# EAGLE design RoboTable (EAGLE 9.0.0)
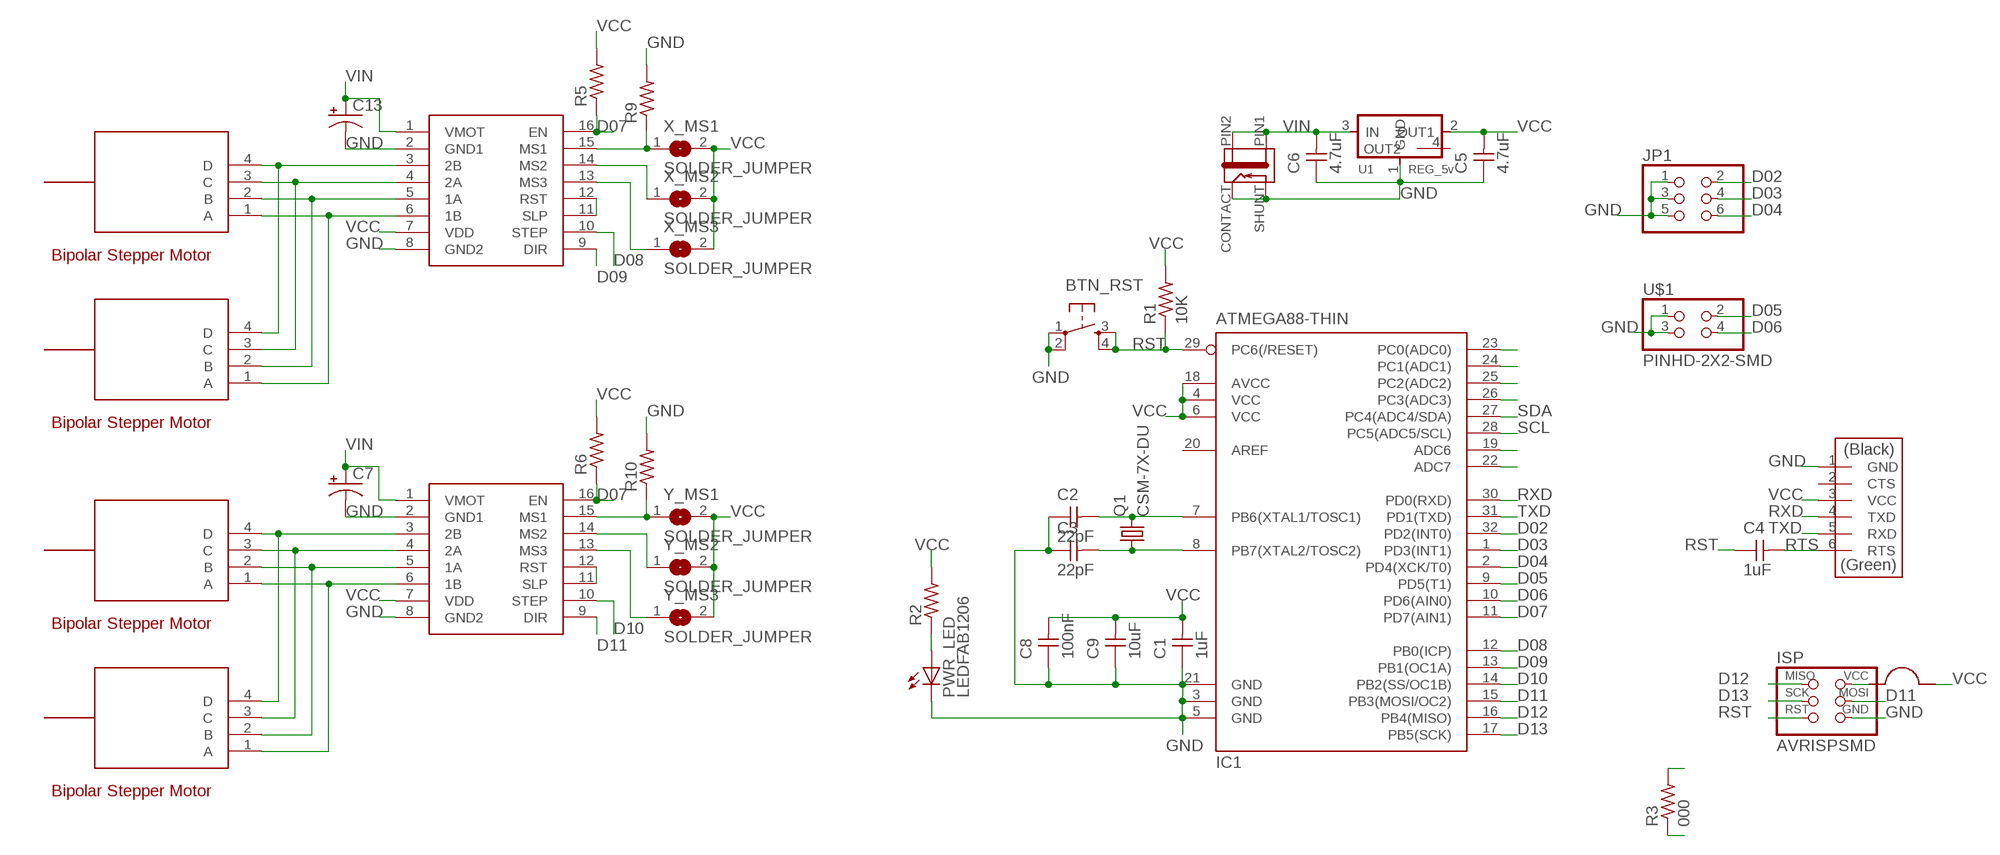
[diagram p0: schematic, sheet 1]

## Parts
BTN_RST  6MM_SWITCH  [6MM_SWITCH_2]
C1  1uF  CAP-UNPOLARIZEDFAB  [C1206FAB]
C2  22pF  CAP-UNPOLARIZEDFAB  [C1206FAB]
C3  22pF  CAP-UNPOLARIZEDFAB  [C1206FAB]
C4  1uF  CAP-UNPOLARIZEDFAB  [C1206FAB]
C5  4.7uF  CAP-UNPOLARIZEDFAB  [C1206FAB]
C6  4.7uF  CAP-UNPOLARIZEDFAB  [C1206FAB]
C7  CPOL-USC  [PANASONIC_C]
C8  100nF  CAP-UNPOLARIZEDFAB  [C1206FAB]
C9  10uF  CAP-UNPOLARIZEDFAB  [C1206FAB]
C13  CPOL-USC  [PANASONIC_C]
FTDI  FTDI-SMD-HEADER  [1X06SMD]
IC1  ATMEGA88-THIN  [TQFP32-08THIN]
ISP  AVRISPSMD  [2X03SMD]
J1  JACK-2.1MM  [PJ-002AH-SMT]
JP1  PINHD-2X3-SMD  [2X03SMD]
PWR_LED  LEDFAB1206  [LED1206FAB]
Q1  CSM-7X-DU  [CSM-7X-DU]
R1  10K  RES-US1206FAB  [R1206FAB]
R2  RES-US1206FAB  [R1206FAB]
R3  000  RES-US1206FAB  [R1206FAB]
R5  RES-US1206FAB  [R1206FAB]
R6  RES-US1206FAB  [R1206FAB]
R9  RES-US1206FAB  [R1206FAB]
R10  RES-US1206FAB  [R1206FAB]
U1  REG_5v  REGULATOR_SOT223  [SOT223]
U$1  PINHD-2X2-SMD  [2X02SMD]
U$4  JUMPER  [JUMPER]
X1_MOTOR  STEPPER_MOTORCONN_1X4  [CONN_1X4]
X2_MOTOR  STEPPER_MOTORCONN_1X4  [CONN_1X4]
X_DRIVER  POLOLUESTEPPERDRIVER  [DIL16]
X_MS1  SOLDER_JUMPER  [SJFAB]
X_MS2  SOLDER_JUMPER  [SJFAB]
X_MS3  SOLDER_JUMPER  [SJFAB]
Y1_MOTOR  STEPPER_MOTORCONN_1X4  [CONN_1X4]
Y2_MOTOR  STEPPER_MOTORCONN_1X4  [CONN_1X4]
Y_DRIVER  POLOLUESTEPPERDRIVER  [DIL16]
Y_MS1  SOLDER_JUMPER  [SJFAB]
Y_MS2  SOLDER_JUMPER  [SJFAB]
Y_MS3  SOLDER_JUMPER  [SJFAB]

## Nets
A_MS1: R9.1 X_DRIVER.15(MS1) X_MS1.1
A_MS2: X_DRIVER.14(MS2) X_MS2.1
A_MS3: X_DRIVER.13(MS3) X_MS3.1
B_MS1: R10.1 Y_DRIVER.15(MS1) Y_MS1.1
B_MS2: Y_DRIVER.14(MS2) Y_MS2.1
B_MS3: Y_DRIVER.13(MS3) Y_MS3.1
D02: IC1.32(PD2(INT0)) JP1.2
D03: IC1.1(PD3(INT1)) JP1.4
D04: IC1.2(PD4(XCK/T0)) JP1.6
D05: IC1.9(PD5(T1)) U$1.2
D06: IC1.10(PD6(AIN0)) U$1.4
D07: IC1.11(PD7(AIN1)) R5.1 R6.1 X_DRIVER.16(EN) Y_DRIVER.16(EN)
D08: IC1.12(PB0(ICP)) X_DRIVER.10(STEP)
D09: IC1.13(PB1(OC1A)) X_DRIVER.9(DIR)
D10: IC1.14(PB2(SS/OC1B)) Y_DRIVER.10(STEP)
D11: IC1.15(PB3(MOSI/OC2)) ISP.4(MOSI) Y_DRIVER.9(DIR)
D12: IC1.16(PB4(MISO)) ISP.1(MISO)
D13: IC1.17(PB5(SCK)) ISP.3(SCK)
GND: BTN_RST.1(P) BTN_RST.2(P1) C1.1 C2.1 C3.1 C5.1 C6.1 C7.- C8.1 C9.1 C13.- FTDI.1(GND) IC1.3(GND) IC1.5(GND) IC1.21(GND) ISP.6(GND) J1.CONTACT J1.SHUNT JP1.1 JP1.3 JP1.5 PWR_LED.2(C) R9.2 R10.2 U1.1(GND) U$1.1 U$1.3 X_DRIVER.2(GND1) X_DRIVER.8(GND2) Y_DRIVER.2(GND1) Y_DRIVER.8(GND2)
LED: PWR_LED.1(A) R2.1
N$1: X_DRIVER.11(SLP) X_DRIVER.12(RST)
N$2: Y_DRIVER.11(SLP) Y_DRIVER.12(RST)
N$3: IC1.23(PC0(ADC0))
N$4: IC1.24(PC1(ADC1))
N$5: IC1.25(PC2(ADC2))
N$6: IC1.26(PC3(ADC3))
N$7: IC1.19(ADC6)
N$8: IC1.22(ADC7)
RST: BTN_RST.3(S) BTN_RST.4(S1) C4.1 IC1.29(PC6(/RESET)) ISP.5(RST) R1.1 R3.1 R3.2
RTS: C4.2 FTDI.6(RTS)
RXD: FTDI.4(TXD) IC1.30(PD0(RXD))
SCL: IC1.28(PC5(ADC5/SCL))
SDA: IC1.27(PC4(ADC4/SDA))
TXD: FTDI.5(RXD) IC1.31(PD1(TXD))
VCC: C1.2 C5.2 C8.2 C9.2 FTDI.3(VCC) IC1.4(VCC) IC1.6(VCC) IC1.18(AVCC) ISP.2(VCC) R1.2 R2.2 R5.2 R6.2 U1.2(OUT1) U$4.P$1 U$4.P$2 X_DRIVER.7(VDD) X_MS1.2 X_MS2.2 X_MS3.2 Y_DRIVER.7(VDD) Y_MS1.2 Y_MS2.2 Y_MS3.2
VIN: C6.2 C7.+ C13.+ J1.PIN1 J1.PIN2 U1.3(IN) X_DRIVER.1(VMOT) Y_DRIVER.1(VMOT)
XA: X1_MOTOR.1(A) X2_MOTOR.1(A) X_DRIVER.6(1B)
XB: X1_MOTOR.2(B) X2_MOTOR.2(B) X_DRIVER.5(1A)
XC: X1_MOTOR.3(C) X2_MOTOR.3(C) X_DRIVER.4(2A)
XD: X1_MOTOR.4(D) X2_MOTOR.4(D) X_DRIVER.3(2B)
XTAL1: C2.2 IC1.7(PB6(XTAL1/TOSC1)) Q1.2
XTAL2: C3.2 IC1.8(PB7(XTAL2/TOSC2)) Q1.1
YA: Y1_MOTOR.1(A) Y2_MOTOR.1(A) Y_DRIVER.6(1B)
YB: Y1_MOTOR.2(B) Y2_MOTOR.2(B) Y_DRIVER.5(1A)
YC: Y1_MOTOR.3(C) Y2_MOTOR.3(C) Y_DRIVER.4(2A)
YD: Y1_MOTOR.4(D) Y2_MOTOR.4(D) Y_DRIVER.3(2B)
Unconnected: FTDI.2(CTS) IC1.20(AREF) U1.4(OUT2)

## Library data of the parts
BTN_RST = fab:6MM_SWITCH: OMRON SWITCH
C1-C6 C8 C9 = fab:CAP-UNPOLARIZED
C7 C13 = rcl:CPOL-US: POLARIZED CAPACITOR, American symbol; SPICEPREFIX: C
FTDI = fab:FTDI-SMD-HEADER
IC1 = fab:ATMEGA88-THIN
ISP = fab:AVRISP
J1 = fab:JACK-2.1MM: SMD DC power jack PJ-002AH-SMT As found in the fablab inventory. Made by Zaerc.
JP1 = fab:PINHD-2X3-SMD: PIN HEADER
PWR_LED = fab:LED: LED
Q1 = crystal:CSM-7X-DU: SMD CRYSTAL; OC_FARNELL: unknown; OC_NEWARK: unknown
R1-R3 R5 R6 R9 R10 = fab:RES-US: Resistor (US Symbol)
U1 = fab:REGULATOR_SOT223
U$1 = fab:PINHD-2X2-SMD
U$4 = fab:JUMPER
X1_MOTOR X2_MOTOR Y1_MOTOR Y2_MOTOR = reprap:STEPPER_MOTOR
X_DRIVER Y_DRIVER = reprap:POLOLUESTEPPERDRIVER: Pololu stepper driver based on the A4983.
X_MS1-X_MS3 Y_MS1-Y_MS3 = fab:SOLDER_JUMPER

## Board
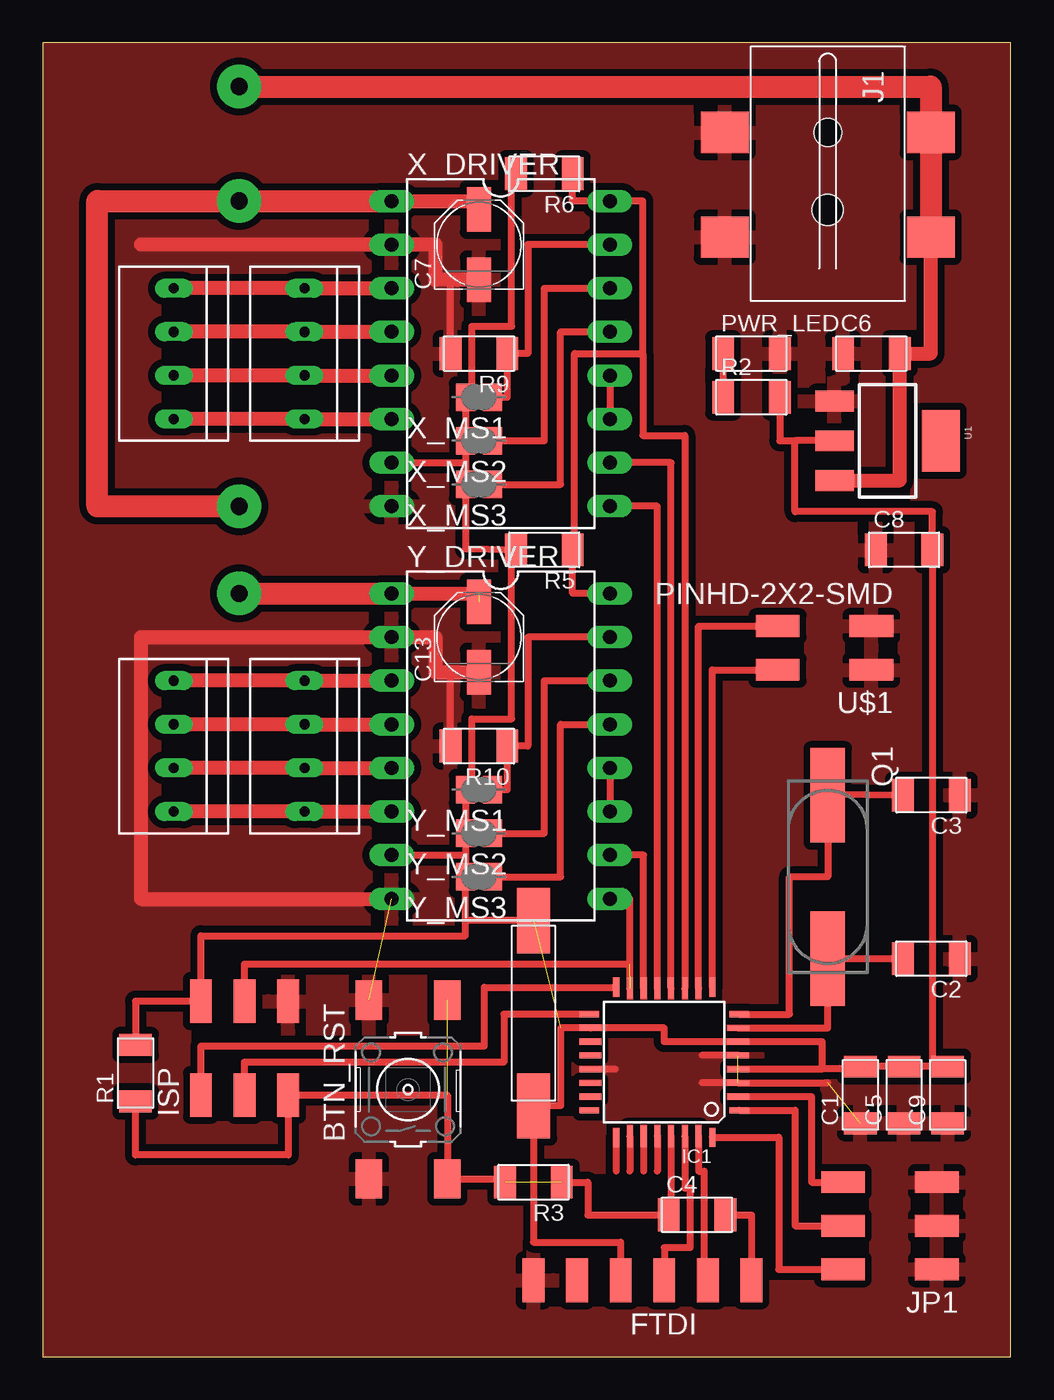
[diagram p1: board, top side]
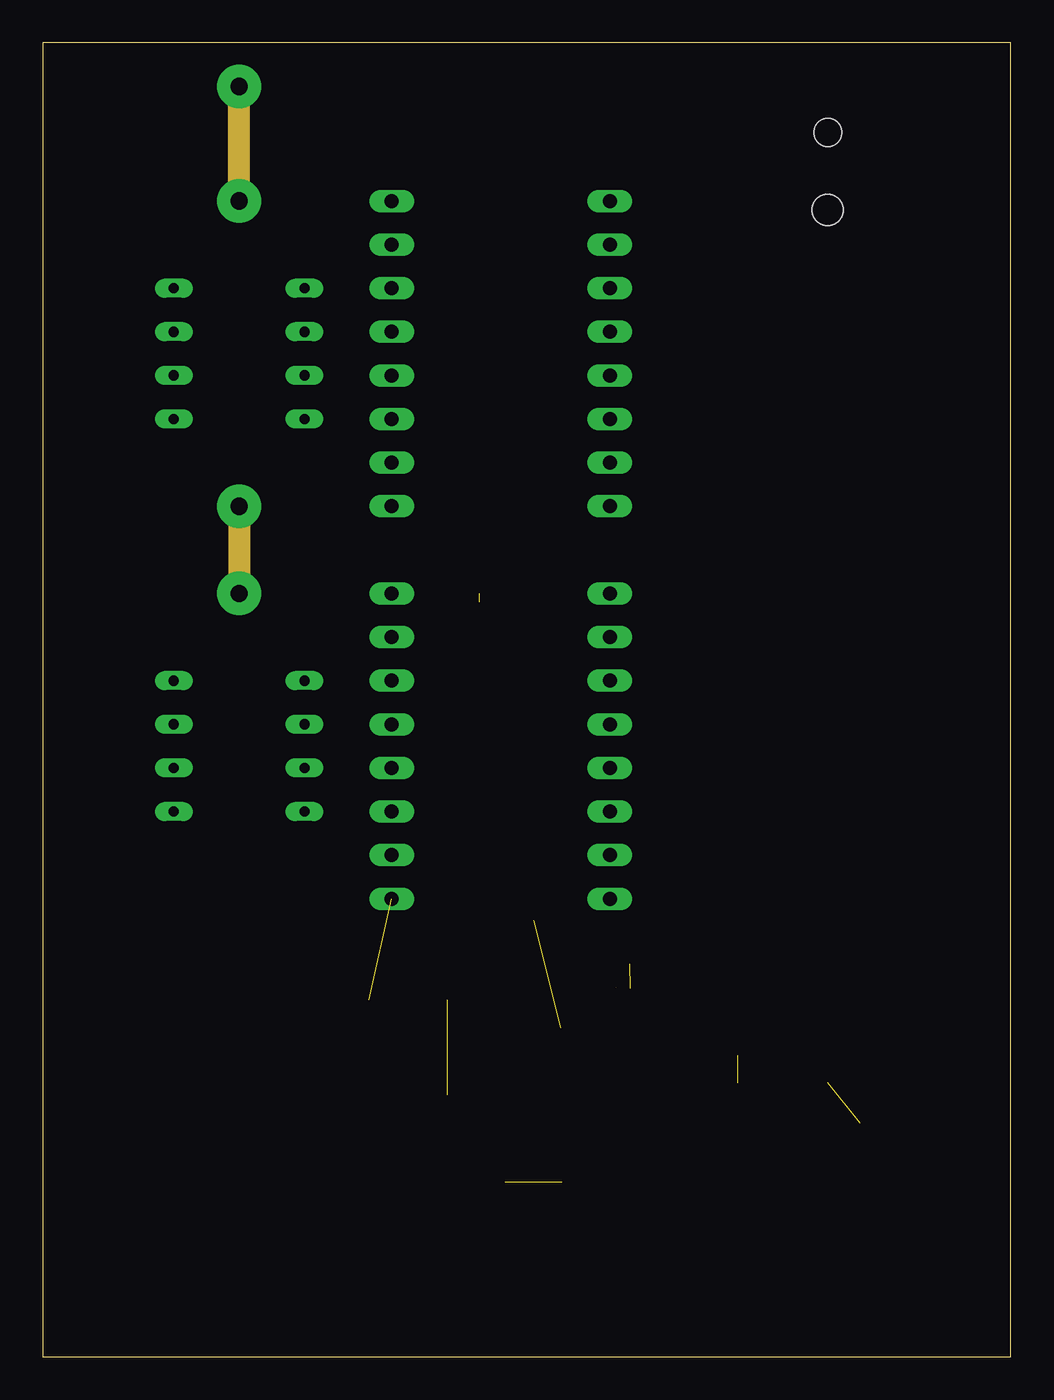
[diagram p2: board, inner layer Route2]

Size 56.39 x 76.52 mm. Coordinates in mm from the lower left corner, seen from the top.
Outline: 0,0 56.39,0 56.39,76.52 0,76.52 0,0
Copper layers (1*2): Top 0.035mm / dielectric 1.5mm / Route2 0.035mm
Design rules "default *": minimum track width 16mil, minimum drill 0.35mm, track to track 16mil, track to pad 16mil, pad to pad 16mil, via to via 16mil, smd to smd 16mil, copper to edge 1mil, drill to drill 16mil, minimum pad ring 10mil, minimum via ring 8mil, stop-mask expansion 0mil, vias tented up to drill 0mil, thermal gap 16mil

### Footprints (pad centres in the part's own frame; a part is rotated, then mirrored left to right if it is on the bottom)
6MM_SWITCH_2 = smd 2.286 x 1.524: 1 -5.207,2.286; 2 5.207,2.286; 3 -5.207,-2.286; 4 5.207,-2.286
C1206FAB = smd 1.27 x 1.905: 1 -1.651,0; 2 1.651,0
PANASONIC_C = smd 2.6 x 1.4: + 2.05,0; - -2.05,0
1X06SMD = smd 2.54 x 1.27: 1 0,6.35; 2 0,3.81; 3 0,1.27; 4 0,-1.27; 5 0,-3.81; 6 0,-6.35
TQFP32-08THIN = smd 1.118 x 0.356: 1 -4.369,2.8; 8 -4.369,-2.8; 17 4.369,-2.8; 24 4.369,2.8 | smd 1.27 x 0.356: 2 -4.293,2; 3 -4.293,1.2; 4 -4.293,0.4; 5 -4.293,-0.4; 6 -4.293,-1.2; 7 -4.293,-2; 18 4.293,-2; 19 4.293,-1.2; 20 4.293,-0.4; 21 4.293,0.4; 22 4.293,1.2; 23 4.293,2 | smd 0.356 x 1.118: 9 -2.8,-4.369; 16 2.8,-4.369; 25 2.8,4.369; 32 -2.8,4.369 | smd 0.356 x 1.27: 10 -2,-4.293; 14 1.2,-4.293; 15 2,-4.293; 26 2,4.293; 27 1.2,4.293; 31 -2,4.293 | smd 0.35 x 1.27: 11 -1.2,-4.293; 12 -0.4,-4.293; 13 0.4,-4.293; 28 0.4,4.293; 29 -0.4,4.293; 30 -1.2,4.293
2X03SMD = smd 2.54 x 1.27: 1 -2.54,2.54; 2 2.92,2.54; 3 -2.54,0; 4 2.92,0; 5 -2.54,-2.54; 6 2.92,-2.54
PJ-002AH-SMT = smd 2.4 x 2.8: CONTACT -2.4,-6; PIN1 3.7,6; PIN2 -2.4,6; SHUNT 3.7,-6 | hole 1.6: -2.4,0 | hole 1.8: 2.1,0
LED1206FAB = smd 1.27 x 1.905: 1 -1.651,0; 2 1.651,0
CSM-7X-DU = smd 5.5 x 2: 1 -4.75,0; 2 4.75,0
R1206FAB = smd 1.27 x 1.905: 1 -1.651,0; 2 1.651,0
SOT223 = smd 1.219 x 2.235: 1 -2.311,-3.099; 2 0,-3.099; 3 2.311,-3.099 | smd 3.6 x 2.2: 4 0,3.099
2X02SMD = smd 2.54 x 1.27: 1 -2.54,1.27; 2 2.92,1.27; 3 -2.54,-1.27; 4 2.92,-1.27
JUMPER = smd 3.81 x 1.93: P$1 -5.397,0; P$2 5.397,0
CONN_1X4 = drill 0.6 long: 1 -3.81,0; 2 -1.27,0; 3 1.27,0; 4 3.81,0
DIL16 = drill 0.813 long: 1 -6.35,15.24; 2 -6.35,12.7; 3 -6.35,10.16; 4 -6.35,7.62; 5 -6.35,5.08; 6 -6.35,2.54; 7 -6.35,0; 8 -6.35,-2.54; 9 6.35,-2.54; 10 6.35,0; 11 6.35,2.54; 12 6.35,5.08; 13 6.35,7.62; 14 6.35,10.16; 15 6.35,12.7; 16 6.35,15.24
SJFAB = smd 1.118 x 1.6: 1 -0.787,0; 2 0.787,0

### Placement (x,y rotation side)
BTN_RST  21.27,15.56 90 top
C1  47.62,15.24 90 top
C2  51.75,23.18 180 top
C3  51.75,32.7 180 top
C4  38.1,8.26 0 top
C5  50.16,15.24 90 top
C6  48.26,58.42 0 top
C7  25.4,64.77 90 top
C8  50.16,46.99 0 top
C9  52.7,15.24 90 top
C13  25.4,41.91 90 top
FTDI  34.92,4.45 90 top
IC1  36.2,17.14 180 top
ISP  11.75,17.78 90 top
J1  45.72,68.9 270 top
JP1  49.53,7.62 180 top
PWR_LED  41.27,58.42 0 top
Q1  45.72,27.94 270 top
R1  5.4,16.51 90 top
R2  41.27,55.88 0 top
R3  28.57,10.16 180 top
R5  29.21,46.99 180 top
R6  29.21,68.9 180 top
R9  25.4,58.42 180 top
R10  25.4,35.56 180 top
U1  49.21,53.34 270 top
U$1  45.72,41.27 180 top
U$4  28.57,20 90 top
X1_MOTOR  15.24,58.42 90 top
X2_MOTOR  7.62,58.42 90 top
X_DRIVER  26.67,52.07 0 top
X_MS1  25.4,55.88 180 top
X_MS2  25.4,53.34 180 top
X_MS3  25.4,50.8 180 top
Y1_MOTOR  15.24,35.56 90 top
Y2_MOTOR  7.62,35.56 90 top
Y_DRIVER  26.67,29.21 0 top
Y_MS1  25.4,33.02 180 top
Y_MS2  25.4,30.48 180 top
Y_MS3  25.4,27.94 180 top

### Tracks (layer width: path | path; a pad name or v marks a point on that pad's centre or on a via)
A_MS1
  Top 0.406: X_DRIVER.15 28.26,64.77 28.26,58.42 R9.1 27.05,55.88 X_MS1.1
A_MS2
  Top 0.406: X_MS2.1 29.21,53.34 29.21,62.23 X_DRIVER.14
A_MS3
  Top 0.406: X_MS3.1 30.16,50.8 30.16,59.69 X_DRIVER.13
B_MS1
  Top 0.406: Y_MS1.1 27.05,33.02 R10.1 28.26,35.56 28.26,41.91 Y_DRIVER.15
B_MS2
  Top 0.406: Y_MS2.1 29.21,30.48 29.21,39.37 Y_DRIVER.14
B_MS3
  Top 0.406: Y_MS3.1 30.16,27.94 30.16,36.83 Y_DRIVER.13
D02
  Top 0.406: IC1.32 42.86,12.78 42.86,5.08 JP1.2
D03
  Top 0.406: IC1.1 43.81,14.35 43.81,7.62 JP1.4
D04
  Top 0.406: IC1.2 44.77,15.14 44.77,10.16 JP1.6
D05
  Top 0.406: IC1.9 38.99,40.01 U$1.2
D06
  Top 0.406: IC1.10 38.2,42.55 U$1.4
D07
  Top 0.406: R6.1 30.86,67.31 X_DRIVER.16 34.95,67.31 34.95,58.42 | Y_DRIVER.16 30.86,44.45 30.86,46.67 | 30.86,46.67 R5.1 | 34.95,58.42 30.98,58.42 30.98,46.67 30.86,46.67 | IC1.11 37.4,53.66 34.95,53.66 34.95,58.42
D08
  Top 0.406: IC1.12 36.59,52.07 X_DRIVER.10
D09
  Top 0.406: IC1.13 35.8,49.53 X_DRIVER.9
D10
  Top 0.406: IC1.14 34.99,29.21 Y_DRIVER.10
D11  (1 unrouted)
  Top 0.406: IC1.15 34.2,26.67 Y_DRIVER.9 | ISP.4 11.75,22.86 34.18,22.86
D12  (1 unrouted)
  Top 0.406: ISP.1 9.21,18.1 25.72,18.1 25.72,21.51 33.38,21.51
D13
  Top 0.406: ISP.3 11.75,17.14 26.85,17.14 26.85,19.95 IC1.17
GND  (3 unrouted)
  Top 0.406: R10.2 23.75,39.86 24.13,39.86 | R9.2 23.75,62.72 24.13,62.72 | IC1.5 38.42,17.55 | 38.42,15.95 IC1.3 45.72,15.95 | IC1.21 33.34,16.75
  Top 0.813: C7.- 24.13,62.72 22.86,62.72 22.86,64.77 X_DRIVER.2 5.7,64.77 | Y_DRIVER.8 5.7,26.67 5.7,41.91 Y_DRIVER.2 22.86,41.91 22.86,39.86 24.13,39.86 C13.-
  pour Top: 0.32,76.2 56.2,76.2 56.2,0 0,0 0,76.2
LED
  Top 0.406: PWR_LED.1 R2.1
N$1
  Top 0.406: X_DRIVER.12 X_DRIVER.11
N$2
  Top 0.406: Y_DRIVER.12 Y_DRIVER.11
N$5
  Top 0.406: IC1.25 33.4,10.79
N$6
  Top 0.406: IC1.26 34.2,10.79
RST  (2 unrouted)
  Top 0.406: R1.1 5.4,11.75 14.29,11.75 ISP.5 23.56,15.24 BTN_RST.3 26.92,10.35 R3.2 | IC1.29 36.59,8.26 C4.1 31.75,8.26 31.75,10.16 R3.1
RTS
  Top 0.406: C4.2 41.27,8.26 FTDI.6
RXD
  Top 0.406: IC1.30 37.4,9.82 37.69,9.82 37.69,6.35 36.2,6.35 FTDI.4
SCL
  Top 0.406: IC1.28 35.8,10.79
SDA
  Top 0.406: IC1.27 34.99,10.79
TXD
  Top 0.406: IC1.31 38.2,10.79 38.51,10.79 38.51,4.36 FTDI.5
VCC  (1 unrouted)
  Top 0.406: 24.61,29.21 Y_MS2.2 Y_MS1.2 24.99,33.02 24.99,37.15 27.3,37.15 27.3,46.99 | 24.61,29.21 Y_MS3.2 24.61,25.4 | Y_DRIVER.7 24.61,29.21 | 24.61,52.07 X_MS2.2 X_MS1.2 24.99,55.88 24.99,60.01 27.3,60.01 27.3,68.9 R6.2 | 24.61,52.07 X_MS3.2 24.61,47.05 27.3,46.99 | X_DRIVER.7 24.61,52.07 | 27.3,46.99 R5.2 | 24.61,25.4 24.61,24.51 9.21,24.51 ISP.2 5.4,20.7 R1.2 | 27.3,46.99 | IC1.4 43.18,16.75 | 43.18,16.75 43.98,16.76 45.4,16.76 | 45.4,16.76 45.4,18.34 IC1.6 36.2,18.34 36.2,19.14 IC1.18 30.16,19.14 30.16,14.61 U$4.P$1 28.57,6.67 33.66,6.67 FTDI.3 | 51.82,16.89 C5.2 C1.2 47.62,16.76 45.4,16.76 | U1.2 43.81,53.34 | 43.81,53.34 43.81,49.21 51.82,49.21 C8.2 51.82,16.89 | R2.2 42.93,53.34 43.81,53.34 | 43.18,16.75 | 51.82,16.89 C9.2 | U$4.P$2 24.61,25.4
VIN  (via drill 1 pad 2.54 layers 1-2)  (1 unrouted)
  Top 0.813: X_DRIVER.1 24.91,67.31 C7.+ | Y_DRIVER.1 25.4,44.45 | U1.3 49.91,51.03 C6.2 51.72,58.42 J1.PIN1
  Top 1.27: J1.PIN1 J1.PIN2 51.72,73.98 v11.43,73.98 | v11.43,49.53 3.17,49.53 3.17,67.31 v11.43,67.31 X_DRIVER.1 | v11.43,44.45 Y_DRIVER.1
  Route2 1.27: v11.43,49.53 v11.43,44.45 | v11.43,67.31 v11.43,73.98
XA
  Top 0.813: X_DRIVER.6 X1_MOTOR.1 X2_MOTOR.1
XB
  Top 0.813: X_DRIVER.5 X1_MOTOR.2 X2_MOTOR.2
XC
  Top 0.813: X_DRIVER.4 X1_MOTOR.3 X2_MOTOR.3
XD
  Top 0.813: X_DRIVER.3 X1_MOTOR.4 X2_MOTOR.4
XTAL1
  Top 0.406: IC1.7 45.72,19.14 Q1.2 49.85,23.19 C2.2
XTAL2
  Top 0.406: C3.2 45.72,32.77 Q1.1 45.72,27.94 43.5,27.94 43.5,19.95 IC1.8
YA
  Top 0.813: Y_DRIVER.6 Y1_MOTOR.1 Y2_MOTOR.1
YB
  Top 0.813: Y_DRIVER.5 Y1_MOTOR.2 Y2_MOTOR.2
YC
  Top 0.813: Y_DRIVER.4 Y1_MOTOR.3 Y2_MOTOR.3
YD
  Top 0.813: Y_DRIVER.3 Y1_MOTOR.4 Y2_MOTOR.4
